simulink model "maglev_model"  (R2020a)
settings: Solver=ode45  StartTime=0.0  StopTime=10.0  RelTol=1e-3  EnableMultiTasking=on
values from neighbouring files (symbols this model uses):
  C = 6.3000e-04    (= 0.00063)    [maglev_init.m]
  g = 9.80    (= 9.8)    [maglev_init.m]
  L1 = 0.6000    (= 0.6)    [maglev_init.m]
  m = 0.0300    (= 0.03)    [maglev_init.m]
  R = 45    [maglev_init.m]
  x1_0 = 0.1    [maglev_init.m]
  x2_0 = 0    [maglev_init.m]
  x3_0 = 0.2    [maglev_init.m]

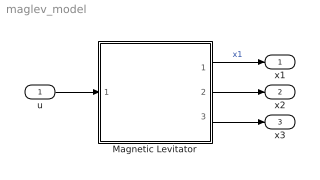
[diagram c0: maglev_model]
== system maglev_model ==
  u : Inport
  Magnetic Levitator : Subsystem  mask{m=m, R=R, L1=L1, C=C, g=g}
      mask prompts: m "ball's mass (m)"; R "Electromagnet's resistance (R)"; L1 "Electromagnet's inductance (L1)"; C "Magnetic force constant (C)"; g "Gravitational acceleration (g)"
  x1 : Outport
  x2 : Outport  Port=2
  x3 : Outport  Port=3
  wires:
  u/1 -> Magnetic Levitator/1(u)
  Magnetic Levitator/1(x1) -> x1/1  "x1"
  Magnetic Levitator/2(x2) -> x2/1
  Magnetic Levitator/3(x3) -> x3/1

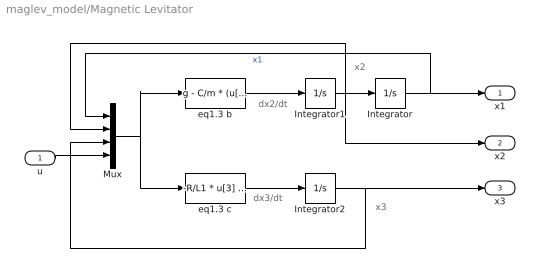
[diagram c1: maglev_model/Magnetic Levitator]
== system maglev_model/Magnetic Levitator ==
  note: x2
  note: x3
  note: dx2/dt
  note: dx3/dt
  u : Inport
  Integrator : Integrator  InitialCondition=x1_0
  Integrator1 : Integrator  InitialCondition=x2_0
  Integrator2 : Integrator  InitialCondition=x3_0
  Mux : Mux
  eq1.3 b : Fcn  Expr=g - C/m * (u[3] / u[1])^2
  eq1.3 c : Fcn  Expr=-R/L1 * u[3] + (2*C)/L1 * ( u[2] * u[3] / u[1]^2 ) + 1/L1 * u[4]
  x1 : Outport
  x2 : Outport  Port=2
  x3 : Outport  Port=3
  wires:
  eq1.3 b/1 -> Integrator1/1
  Integrator1/1 -> Integrator/1, Mux/2, x2/1
  eq1.3 c/1 -> Integrator2/1
  Mux/1 -> eq1.3 b/1, eq1.3 c/1
  Integrator/1 -> Mux/1, x1/1  "x1"
  Integrator2/1 -> Mux/3, x3/1
  u/1 -> Mux/4
